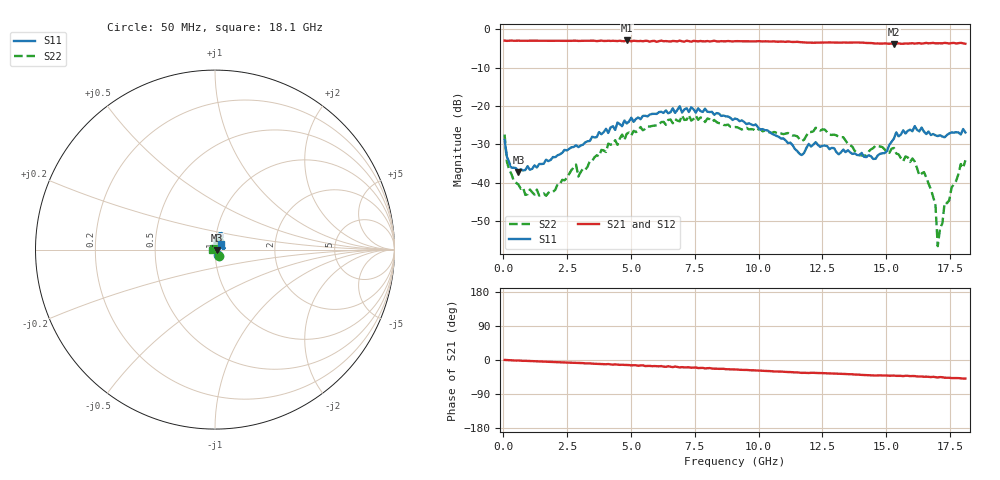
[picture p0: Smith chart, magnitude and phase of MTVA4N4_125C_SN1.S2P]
! Network Analyzer HP8720D.06.14 Serial No. US36140669
! 28 Jun 2005  10:31:56
! Frequency  S11  S21  S12  S22
# HZ  S  DB R 50
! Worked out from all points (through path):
!   201 points, 50 MHz to 18.1 GHz, reference 50 ohm
!   highest |S21| = -2.95 dB at 4.833 GHz (marker M1); lowest = -3.8 dB at 15.3 GHz (marker M2)
!   group delay of S21, straight-line fit = 7.57 ps
!   lowest |S11| = -37.2 dB at 591.5 MHz (marker M3), VSWR 1.03, Z = 51.3 - j0.45 ohm
!   |S11| at or under -10 dB: start of sweep to end of sweep
!   |S22| runs from -56.4 to -22.4 dB; largest |S21 - S12| = 0.02
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5e7  -28.77 -59.6  -2.98 0.2  -3.00 0.3  -27.43 -55.9
1.4025e8  -33.20 -45.5  -3.06 -0.2  -3.05 -0.2  -34.51 -56.2
5.915e8  -37.18 -18.5  -3.00 -1.4  -3.04 -1.4  -40.44 -27.5
1.6745e9  -33.95 0.4  -3.03 -4.4  -3.03 -4.5  -43.35 10.9
2.84775e9  -30.21 22.3  -3.02 -7.9  -3.03 -7.8  -35.23 59.2
3.1185e9  -30.05 30.4  -3.02 -8.2  -3.05 -8.5  -36.30 71.6
4.83325e9  -24.53 57.8  -2.95 -13.1  -3.04 -13.4  -27.20 67.9
6.09675e9  -21.58 61.5  -3.12 -16.7  -3.05 -16.6  -24.80 68.4
7.27e9  -21.56 69.7  -3.14 -19.2  -3.18 -20.5  -22.38 65.1
9.075e9  -23.26 84.1  -3.14 -25.0  -3.13 -25.1  -25.46 48.1
1.169225e10  -32.75 100.3  -3.42 -34.0  -3.42 -33.9  -29.11 64.6
1.21435e10  -30.02 86.9  -3.55 -33.7  -3.51 -33.9  -26.58 77.5
1.331675e10  -31.32 44.2  -3.48 -36.6  -3.49 -36.9  -28.11 85.6
1.39485e10  -32.77 1.3  -3.51 -38.8  -3.49 -39.0  -32.81 115.1
1.449e10  -33.76 -1.6  -3.70 -40.6  -3.72 -40.8  -30.96 137.2
1.512175e10  -30.09 22.3  -3.80 -41.5  -3.73 -41.3  -32.18 134.5
1.530225e10  -28.44 12.9  -3.85 -41.1  -3.74 -42.1  -30.91 133.3
1.64755e10  -26.66 15.1  -3.69 -44.3  -3.82 -43.3  -37.18 57.2
1.692675e10  -27.61 24.1  -3.70 -45.0  -3.59 -45.0  -45.71 4.2
1.7017e10  -27.82 25.8  -3.69 -46.0  -3.78 -46.6  -56.45 30.3
1.728775e10  -28.12 36.1  -3.58 -46.8  -3.55 -46.7  -45.10 -135.7
1.81e10  -26.90 46.8  -3.81 -49.0  -3.80 -49.9  -34.11 -169.8
